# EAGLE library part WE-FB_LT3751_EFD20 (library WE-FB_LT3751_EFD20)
Flyback Converter WE-FB for LT3751 - designd for LT3751
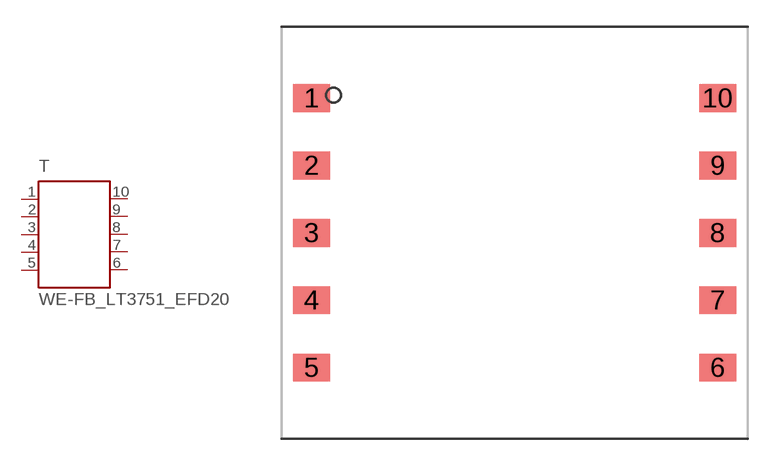
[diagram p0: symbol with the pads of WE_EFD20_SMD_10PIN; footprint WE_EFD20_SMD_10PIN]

Designator prefix T

## WE-FB_LT3751_EFD20-750032051 (MPN: 750032051; OC_FARNELL: 1748692; OC_NEWARK: 34R6105; PACKAGE: EFD20_SMD_10PIN; SUPPLIER: Würth Elektronik eiSos GmbH), WE-FB_LT3751_EFD20-750032052 (MPN: 750032052; OC_FARNELL: 1748693; OC_NEWARK: 34R6106; PACKAGE: EFD20_SMD_10PIN; SUPPLIER: Würth Elektronik eiSos GmbH)  [WE_EFD20_SMD_10PIN]
1  1  pas
2  2  pas
3  3  pas
4  4  pas
5  5  pas
6  6  pas
7  7  pas
8  8  pas
9  9  pas
10  10  pas

## Footprint WE_EFD20_SMD_10PIN (pad centres in mm)
Transformer, EFD20 SMD 10 Pin
smd 2.08 x 1.55: 1 -11.33,7.52; 2 -11.33,3.76; 3 -11.33,0; 4 -11.33,-3.76; 5 -11.33,-7.52; 6 11.33,-7.52; 7 11.33,-3.76; 8 11.33,0; 9 11.33,3.76; 10 11.33,7.52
